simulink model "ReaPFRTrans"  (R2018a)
settings: Solver=VariableStepAuto  StartTime=0.0  StopTime=25  RelTol=1e-3
undefined symbols (not defined in the file): a402, ReaPFRTrans, sdiscope

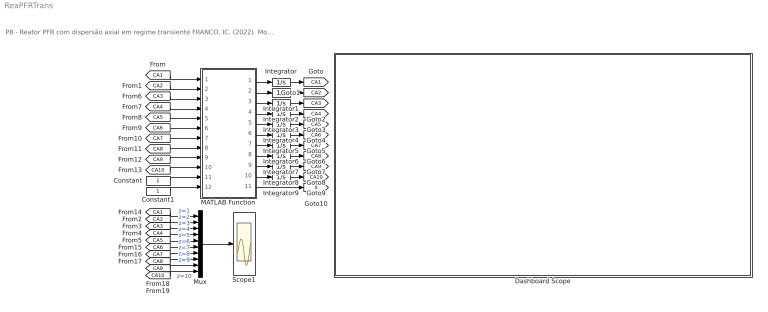
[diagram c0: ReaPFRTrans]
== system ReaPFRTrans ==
  note: P8 - Reator PFR com dispersão axial em regime transiente FRANCO, IC. (2022). Modelagem e Simulação: Problemas Típicos da Engenharia Química para Simulação e Análise. NOTAS DE AULA INOVADORAS. The Journal of Engineering and Exact Sciences. Material Complementar.
  Constant : Constant
  Constant1 : Constant
  Dashboard Scope : Subsystem  DialogController=hmiCreateDDGDialog  IsWebBlock=on  mask(MWDashboardBlock){webBlockId=5ac27d2b-88ae-4a21-a402-8647a1864648, webBlockType=sdiscope, ShowInitialText=on, HMISrcModelName=ReaPFRTrans}
      mask prompts: webBlockId "WebBlock Id"; webBlockType "WebBlock Type"; HMISrcModelName "Source Model"
      mask help: SimulinkHMI:dialogs:HMIScopeDialogDesc
  Integrator{,1..9} (10 alike) : Integrator
  MATLAB Function : MATLAB Function  TreatAsAtomicUnit=on
  Mux : Mux  Inputs=10
  Scope1 : Scope
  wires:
  Integrator3/1 -> [CA4]
  MATLAB Function/4(dC4) -> Integrator3/1
  Integrator1/1 -> [CA2]
  [CA9] -> MATLAB Function/9(C9)
  MATLAB Function/11(X) -> [X]
  Integrator4/1 -> [CA5]
  MATLAB Function/5(dC5) -> Integrator4/1
  MATLAB Function/9(dC9) -> Integrator8/1
  Constant1/1 -> MATLAB Function/12(u)
  [CA4] -> MATLAB Function/4(C4)
  Integrator2/1 -> [CA3]
  [CA8] -> MATLAB Function/8(C8)
  [CA5] -> MATLAB Function/5(C5)
  [CA7] -> MATLAB Function/7(C7)
  MATLAB Function/3(dC3) -> Integrator2/1
  MATLAB Function/2(dC2) -> Integrator1/1
  [CA3] -> MATLAB Function/3(C3)
  Constant/1 -> MATLAB Function/11(CA0)
  [CA1] -> MATLAB Function/1(C1)
  MATLAB Function/7(dC7) -> Integrator6/1
  Integrator6/1 -> [CA7]
  MATLAB Function/10(dC10) -> Integrator9/1
  [CA2] -> MATLAB Function/2(C2)
  Integrator7/1 -> [CA8]
  Integrator9/1 -> [CA10]
  Integrator5/1 -> [CA6]
  Integrator/1 -> [CA1]
  MATLAB Function/6(dC6) -> Integrator5/1
  MATLAB Function/8(dC8) -> Integrator7/1
  Integrator8/1 -> [CA9]
  [CA6] -> MATLAB Function/6(C6)
  [CA10] -> MATLAB Function/10(C10)
  MATLAB Function/1(dC1) -> Integrator/1
  [CA1] -> Mux/1  "z=1"
  [CA2] -> Mux/2  "z=2"
  [CA3] -> Mux/3  "z=3"
  [CA4] -> Mux/4  "z=4"
  [CA5] -> Mux/5  "z=5"
  [CA6] -> Mux/6  "z=6"
  [CA7] -> Mux/7  "z=7"
  [CA8] -> Mux/8  "z=8"
  [CA9] -> Mux/9  "z=9"
  [CA10] -> Mux/10  "z=10"
  Mux/1 -> Scope1/1

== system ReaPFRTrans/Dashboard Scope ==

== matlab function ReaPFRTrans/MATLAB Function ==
function [dC1,dC2,dC3,dC4,dC5,dC6,dC7,dC8,dC9,dC10,X] = fcn(C1,C2,C3,C4,C5,C6,C7,C8,C9,C10,CA0,u)
%% Parâmetros
D =  1.00;
k =  0.03;
L = 10.00;
N = 10.00;

%% equações auxiliares
dz= L/N;

%conversão
X=[(CA0-C1)/CA0;
   (CA0-C2)/CA0;
   (CA0-C3)/CA0;
   (CA0-C4)/CA0;
   (CA0-C5)/CA0;
   (CA0-C6)/CA0;
   (CA0-C7)/CA0;
   (CA0-C8)/CA0;
   (CA0-C9)/CA0;
   (CA0-C10)/CA0];

%% Modelo matemático
dC1 = u*(CA0-C1)/dz+D*(CA0-2*C1+C2)/dz^2-k*C1;
dC2 = u*(C1-C2)/dz+D*(C1-2*C2+C3)/dz^2-k*C2;
dC3 = u*(C2-C3)/dz+D*(C2-2*C3+C4)/dz^2-k*C3;
dC4 = u*(C3-C4)/dz+D*(C3-2*C4+C5)/dz^2-k*C4;
dC5 = u*(C4-C5)/dz+D*(C4-2*C5+C6)/dz^2-k*C5;
dC6 = u*(C5-C6)/dz+D*(C5-2*C6+C7)/dz^2-k*C6;
dC7 = u*(C6-C7)/dz+D*(C6-2*C7+C8)/dz^2-k*C7;
dC8 = u*(C7-C8)/dz+D*(C7-2*C8+C9)/dz^2-k*C8;
dC9 = u*(C8-C9)/dz+D*(C8-2*C9+C10)/dz^2-k*C9;
dC10= u*(C9-C10)/dz+D*(C9-2*C10+C10)/dz^2-k*C10;
end
